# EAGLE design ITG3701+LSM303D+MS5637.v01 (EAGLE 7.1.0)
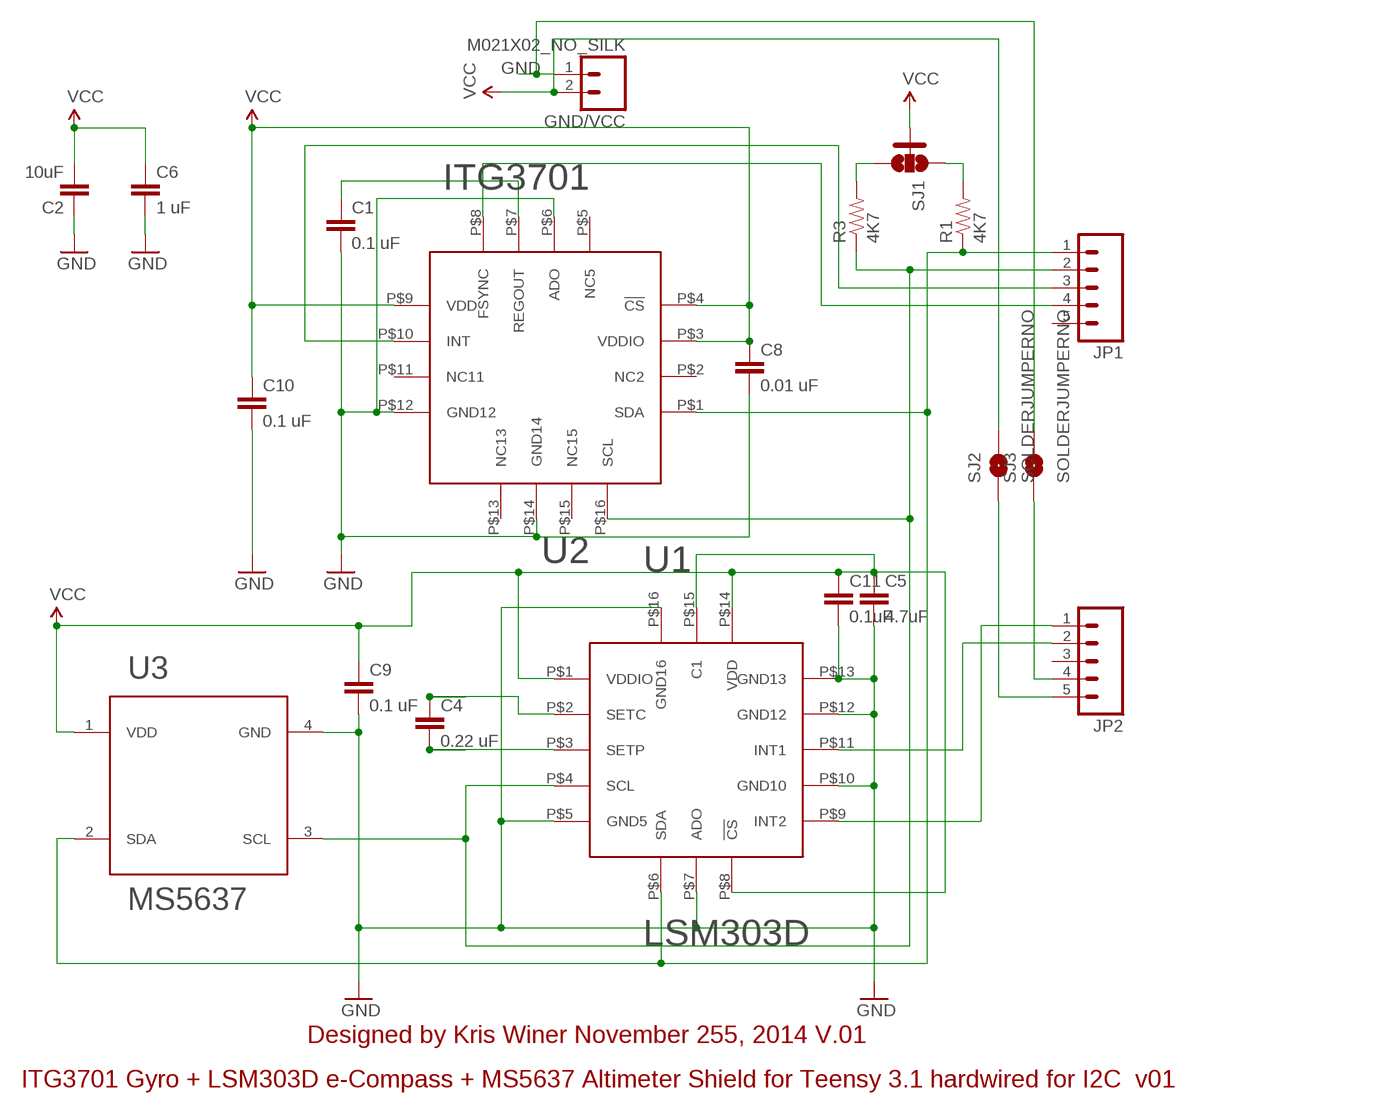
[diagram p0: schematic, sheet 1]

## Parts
C1  0.1 uF  CAP0402-CAP  [0402-CAP]
C2  10uF  0.22UF-25V-10%(0603)  [0603-CAP]
C4  0.22 uF  CAP0402-CAP  [0402-CAP]
C5  4.7uF  CAP0402-CAP  [0402-CAP]
C6  1 uF  CAP0402-CAP  [0402-CAP]
C8  0.01 uF  CAP0402-CAP  [0402-CAP]
C9  0.1 uF  CAP0402-CAP  [0402-CAP]
C10  0.1 uF  CAP0402-CAP  [0402-CAP]
C11  0.1uF  CAP0402-CAP  [0402-CAP]
GND/VCC  M021X02_NO_SILK  [1X02_NO_SILK]
JP1  M05NO_SILK  [1X05_NO_SILK]
JP2  M05NO_SILK  [1X05_NO_SILK]
R1  4K7  RESISTOR0402-RES  [0402-RES]
R3  4K7  RESISTOR0402-RES  [0402-RES]
SJ1  SOLDERJUMPER_2WAYS  [SJ_3]
SJ2  SOLDERJUMPERNO  [SJ_2S-NO]
SJ3  SOLDERJUMPERNO  [SJ_2S-NO]
U1  LSM303D  [LSM303D]
U2  ITG3701  [ITG3701-QFN16]
U3  MS5637  [MS5637QFN-4]

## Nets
GND: C1.2 C2.1 C5.2 C6.2 C8.2 C9.2 C10.2 C11.2 GND/VCC.1 SJ3.2 U1.P$5(GND5) U1.P$7(ADO) U1.P$10(GND10) U1.P$12(GND12) U1.P$13(GND13) U1.P$16(GND16) U2.P$6(ADO) U2.P$12(GND12) U2.P$14(GND14) U3.4(GND)
N$2: JP2.4 SJ3.1
N$3: C4.2 U1.P$3(SETP)
N$4: C4.1 U1.P$2(SETC)
N$5: JP2.2 U1.P$11(INT1)
N$6: JP2.1 U1.P$9(INT2)
N$7: JP1.2 R3.1 U1.P$4(SCL) U2.P$16(SCL) U3.3(SCL)
N$8: JP1.3 U2.P$10(INT)
N$9: R3.2 SJ1.3
N$10: R1.2 SJ1.1
N$11: C1.1 U2.P$7(REGOUT)
N$12: U1.P$15(C1)
N$13: JP2.5 SJ2.1
N$15: JP1.4 U2.P$8(FSYNC)
SDO: JP1.1 R1.1 U1.P$6(SDA) U2.P$1(SDA) U3.2(SDA)
VCC: C2.2 C5.1 C6.1 C8.1 C9.1 C10.1 C11.1 GND/VCC.2 SJ1.2 SJ2.2 U1.P$1(VDDIO) U1.P$8(!CS) U1.P$14(VDD) U2.P$3(VDDIO) U2.P$4(!CS) U2.P$9(VDD) U3.1(VDD)
Unconnected: JP1.5 JP2.3 U2.P$2(NC2) U2.P$5(NC5) U2.P$11(NC11) U2.P$13(NC13) U2.P$15(NC15)

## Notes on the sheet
- Designed by Kris Winer November 255, 2014 V.01
- ITG3701 Gyro + LSM303D e-Compass + MS5637 Altimeter Shield for Teensy 3.1 hardwired for I2C  v01

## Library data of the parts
C1 C4-C6 C8-C11 = SparkFun-Capacitors:CAP: Capacitor
C2 = SparkFun-Capacitors:0.22UF-25V-10%(0603): CAP-07822; PROD_ID: CAP-07822; VALUE: 0.22uF
GND/VCC = SparkFun-Connectors:M02: Standard 2-pin 0.1" header. Use with
JP1 JP2 = SparkFun-Connectors:M05: Header 5 Standard 5-pin 0.1" header. Use with straight break away headers (SKU : PRT-00116), right angle break away headers (PRT-00553), swiss pins (PRT-00743), machine pins (PRT-00117), and female headers (PRT-00115). Molex polarized connector foot print use with SKU : PRT-08230 with associated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
R1 R3 = SparkFun-Passives:RESISTOR: Resistor
SJ1 = SparkFun-Passives:SOLDERJUMPER_2WAY: Solder Jumper 2 way solder jumper
SJ2 SJ3 = SparkFun-Retired:SOLDERJUMPER: Solder Jumper
U1 = Kris':LSM303D: ST Microelectronics' LSM303D e-compass in LGA-16 package
U2 = Kris':ITG3701: ITG3701 Invensense gyroscope with +/- 4000 dps FS range in QFN-16 package
U3 = SparkFun-DiscreteSemi:MS5637: MS5637 I2C pressure sensor in QFN-4 package by Measurement Specialties

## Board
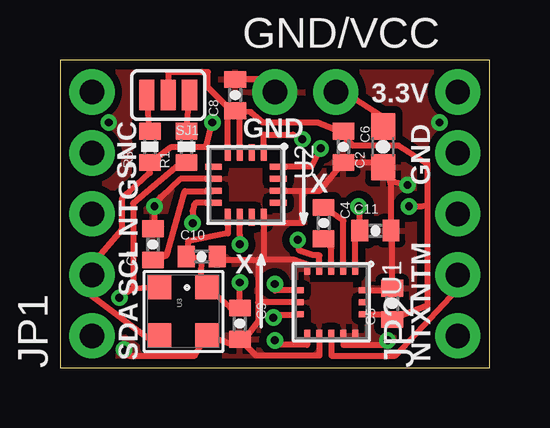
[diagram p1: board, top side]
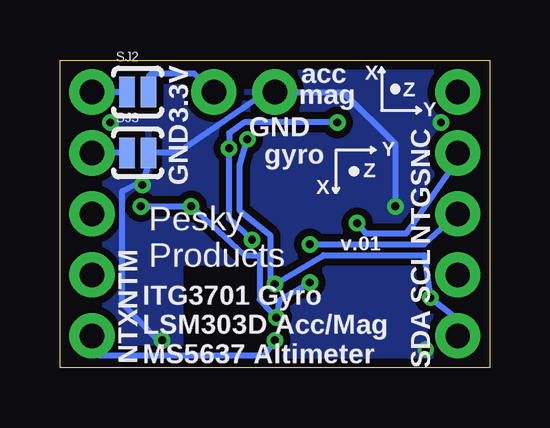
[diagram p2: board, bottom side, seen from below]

Size 17.91 x 12.83 mm. Coordinates in mm from the lower left corner, seen from the top.
Outline: 0,0 17.91,0 17.91,12.83 0,12.83 0,0
Copper layers (1*16): Top 0.0356mm / dielectric 1.5011mm / Bottom 0.0356mm
Design rules "OSHPark *": minimum track width 6mil, minimum drill 13mil, track to track 6mil, track to pad 6mil, pad to pad 6mil, via to via 6mil, smd to smd 6mil, copper to edge 15mil, drill to drill 6mil, minimum pad ring 7mil, minimum via ring 7mil, stop-mask expansion 3mil, vias tented up to drill 20mil, thermal gap 10mil

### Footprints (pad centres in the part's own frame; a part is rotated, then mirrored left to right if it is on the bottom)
0402-CAP = smd 0.7 x 0.9: 1 -0.65,0; 2 0.65,0
0603-CAP = smd 1.1 x 1: 1 -0.85,0; 2 0.85,0
1X02_NO_SILK = drill 1.016 pad 1.88: 1 0,0; 2 2.54,0
1X05_NO_SILK = drill 1.016 pad 1.88: 1 0,0; 2 2.54,0; 3 5.08,0; 4 7.62,0; 5 10.16,0
0402-RES = smd 0.7 x 0.9: 1 -0.65,0; 2 0.65,0
SJ_3 = smd 0.635 x 1.27: 1 -0.889,0; 2 0,0; 3 0.889,0
SJ_2S-NO = smd 0.635 x 1.27: 1 -0.45,0; 2 0.45,0
LSM303D = smd 0.5 x 0.25: P$1 -1.4,1; P$2 -1.4,0.5; P$3 -1.4,0; P$4 -1.4,-0.5; P$5 -1.4,-1; P$9 1.4,-1; P$10 1.4,-0.5; P$11 1.4,0; P$12 1.4,0.5; P$13 1.4,1 | smd 0.25 x 0.5: P$6 -0.5,-1.4; P$7 0,-1.4; P$8 0.5,-1.4; P$14 0.5,1.4; P$15 0,1.4; P$16 -0.5,1.4
ITG3701-QFN16 = smd 0.7 x 0.25: P$1 -1.35,0.75; P$2 -1.35,0.25; P$3 -1.35,-0.25; P$4 -1.35,-0.75; P$9 1.35,-0.75; P$10 1.35,-0.25; P$11 1.35,0.25; P$12 1.35,0.75 | smd 0.25 x 0.7: P$5 -0.75,-1.35; P$6 -0.25,-1.35; P$7 0.25,-1.35; P$8 0.75,-1.35; P$13 0.75,1.35; P$14 0.25,1.35; P$15 -0.25,1.35; P$16 -0.75,1.35
MS5637QFN-4 = smd 1 x 1: 1 -1,1; 2 -1,-1; 3 1,-1; 4 1,1

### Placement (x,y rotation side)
C1  3.87,5.14 90 top
C2  13.46,9.21 90 top
C4  10.99,6.03 270 top
C5  13.84,2.67 90 top
C6  11.81,9.21 270 top
C8  7.3,11.37 90 top
C9  7.49,1.84 270 top
C10  5.91,4.64 0 top
C11  13.14,5.71 0 top
GND/VCC  8.95,11.49 0 top
JP1  1.33,1.33 90 top
JP2  16.57,1.33 90 top
R1  5.27,9.21 90 top
R3  3.75,9.21 90 top
SJ1  4.51,11.37 180 top
SJ2  14.67,11.49 0 bottom
SJ3  14.67,8.95 0 bottom
U1  11.3,2.73 270 top
U2  7.75,7.62 270 top
U3  5.14,2.35 270 top

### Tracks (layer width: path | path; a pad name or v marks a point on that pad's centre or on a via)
GND  (via drill 0.33)
  Top 0.254: U1.P$16 13.76,3.23 C5.2 13.84,5.48 C11.2 13.79,7.6 13.76,7.75 | C9.2 7.08,1.03 U3.4 5.62,0.51 2.86,0.51 v2.67,0.76 | U2.P$12 8.5,6.03 | U2.P$14 10.1,7.37 | 10.1,7.37 10.81,7.37 C6.2 13.39,8.56 C2.1 13.76,7.75 | U2.P$6 5.01,7.87 4.19,7.11 v3.94,6.73 3.94,5.98 C1.2 | U1.P$7 8.26,2.73 | C9.2 7.48,1.33 7.81,1.33 8.26,1.94 8.26,2.73 | 8.5,6.03 10.1,6.03 10.1,7.37 | 8.5,6.03 8.5,4.51 | 8.5,4.51 8.26,4.51 8.26,2.73 | 8.5,4.51 8.08,4.49 6.92,4.49 C10.2 | v14.48,7.62 13.76,7.75 | U1.P$5 10.3,4.3 9.72,4.51 8.5,4.51 | C8.2 8.43,12.02 GND/VCC.1 | U1.P$10 10.8,0.52 10.79,0.51 8.18,0.51 C9.2 | U1.P$12 11.8,1.02 11.81,0.95 12.32,0.95 | 12.32,0.95 13.53,0.95 v13.65,1.14 | U1.P$13 12.3,0.97 12.32,0.95
  Bottom 0.254: SJ3.2 13.97,8.95 | 13.97,8.95 13.02,8.95 9.34,11.49 GND/VCC.1 6.1,11.49 3.94,9.34 v3.94,6.73 | 13.97,8.95 14.22,8.51 v14.48,7.62 14.54,7.68 14.67,7.68 15.3,7.37 15.3,2.67 13.84,1.14 v13.65,1.14
  other vias: 2.03,10.22 15.81,10.22
  pour Top (isolate 0.305): 0.06,12.76 0.06,0 3.49,0 3.49,3.62 6.79,3.62 6.79,3.75 6.86,3.75 6.86,0 17.91,0 17.91,12.76 0.06,12.76
  pour Bottom (isolate 0.305): 0.06,12.83 0.06,0 9.78,0 9.78,4.38 12.89,4.38 12.89,-0.06 17.91,-0.06 17.91,12.83 0.13,12.83
N$2
  Bottom 0.254: SJ3.1 JP2.4
N$3
  Top 0.254: U1.P$3 11.3,5 C4.2
N$4
  Top 0.254: U1.P$2 11.8,6.12 C4.1
N$5
  Top 0.254: U1.P$11 11.3,0.51 13.97,0.51 16.57,3.3 JP2.2
N$6  (via drill 0.33)
  Top 0.254: 10.3,1.01 U1.P$9 10.3,1.03 10.29,0.95 9.08,0.95 v8.95,1.14
  Bottom 0.254: v8.95,1.14 9.4,0.51 16.26,0.51 JP2.1
N$7  (via drill 0.33)
  Top 0.254: v6.35,10.22 6.1,9.21 4.64,9.21 4.11,8.81 R3.1 3.75,8.13 2.91,7.35 2.6,7.1 2.6,5.78 1.33,4.32 JP1.2 1.33,2.98 3.62,1.27 4.13,1.27 U3.3 | v10.86,9.14 10.48,8.38 9.11,8.38 U2.P$16 | U1.P$4 10.8,4.69 10.54,4.7 9.97,4.89 v9.91,5.33
  Bottom 0.254: v9.91,5.33 10.86,6.22 v10.86,9.14 10.86,9.78 10.22,10.22 v6.35,10.22
N$8  (via drill 0.33)
  Top 0.254: v7.49,5.14 7.5,5.53 U2.P$10
  Bottom 0.254: v7.49,5.14 2.73,5.14 JP1.3
N$9
  Top 0.254: R3.2 SJ1.3
N$10
  Top 0.254: R1.2 SJ1.1
N$11
  Top 0.254: C1.1 4.45,4.7 5.21,7.37 U2.P$7
N$13
  Bottom 0.254: SJ2.1 JP2.5
N$15  (via drill 0.33)
  Top 0.254: U2.P$8 5.66,6.87 5.59,6.79 5.52,6.54 v5.52,6.03
  Bottom 0.254: JP1.4 1.27,8.89 1.27,8.76 3.17,6.03 3.49,5.59 5.14,5.59 v5.52,6.03
SDO  (via drill 0.33)
  Top 0.254: U3.2 3.05,3.29 | 3.05,3.29 2.62,3.03 v2.48,2.92 | R1.1 5.07,8.56 3.05,6.86 3.05,3.29 | U1.P$6 8.96,3.23 v8.95,3.49 | U2.P$1 8.5,9.7 8.51,9.72 9.72,9.72 v10.1,9.53
  Bottom 0.254: JP1.1 1.33,2.03 v2.48,2.92 2.73,4.7 6.92,4.7 v8.95,3.49 9.14,3.68 9.14,5.52 10.41,6.54 10.41,8.45 v10.1,9.53
VCC  (via drill 0.33)
  Top 0.254: U1.P$14 13.82,2.23 C5.1 15.3,2.59 15.3,6.79 | SJ1.2 4.51,12.32 6.16,12.32 6.16,11.68 7.19,10.65 C8.1 | U2.P$9 7,5.6 5.33,5.27 5.27,4.46 C10.1 5.51,4.57 5.91,4.57 5.89,3.83 U3.1 7.08,2.52 C9.1 v7.49,3.56 | GND/VCC.2 11.87,11.49 13.53,10.41 C2.2 13.46,9.34 13.4,9.27 | v8.89,2.1 8.89,2.22 U1.P$8 | C8.1 7.95,10.65 8.45,10.22 10.73,10.22 11.41,9.97 C6.1 11.95,10.06 11.95,9.52 12.19,9.27 13.4,9.27 | C8.1 7,10.41 U2.P$4 | U2.P$3 7.5,10.46 C8.1 | 13.4,9.27 14.1,9.27 15.3,8.51 15.3,6.79 | v14.54,6.73 15.05,6.73 15.3,6.79 | U1.P$1 12.3,5.46 C11.1 12.49,6.49 v12.45,6.73
  Bottom 0.254: v7.49,3.56 8.76,2.79 v8.89,2.1 9.59,2.86 9.59,4.7 10.22,4.7 v12.45,6.73 v14.54,6.73 | GND/VCC.2 11.56,11.49 12.32,12.26 14.1,12.26 14.22,12.13 SJ2.2

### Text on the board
tPlace: 3.3V | GND | GND | SNC | X | NTG | X | SCL | NTM | SDA | NTX
bPlace: X | mag | acc | Z | Y | SNC | GND | 3.3V | GND | Y | gyro | NTG | Z | X | SCL | v.01 | NTM | Pesky / Products | SDA | NTX | ITG3701 Gyro / LSM303D Acc/Mag / MS5637 Altimeter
